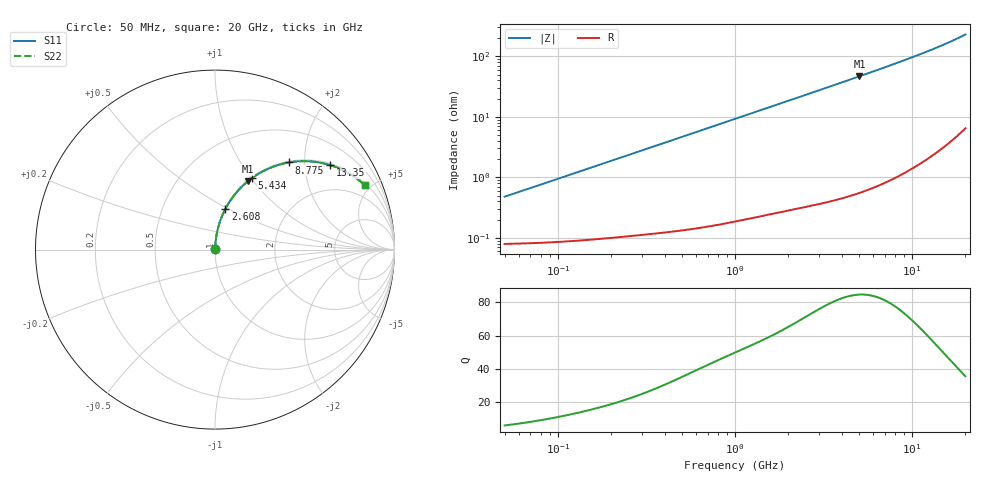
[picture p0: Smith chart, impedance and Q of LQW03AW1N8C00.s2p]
!Murata Part Number: LQW03AW1N8C00
!These Parameters are Measured in Series Mode Connection
!  o--[Z]--o
!Port1  Port2
!  o-------o
!Freq. Start=50[MHz] Stop=20[GHz], 401[Steps]
# Hz S RI R 50
!Freq.(Hz) S11(Real) S11(Imag) S21(Real) S21(Imag) S12(Real) S12(Imag) S22(Real) S22(Imag)
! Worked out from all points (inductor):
!   401 points, 50 MHz to 20 GHz, reference 50 ohm
!   read as one part in series: L = 1.5 nH near 51.52 MHz
!   highest Q = 84.6 at 5.041 GHz (marker M1), where L = 1.48 nH
!   S11 on the Smith chart (normalised r, x): 50 MHz: 1.00, +0.01; 2.608 GHz: 1.01, +0.48; 5.434 GHz: 1.01, +1.01; 8.775 GHz: 1.02, +1.67; 13.35 GHz: 1.05, +2.69; 20 GHz: 1.13, +4.60
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5e7  0.000816 0.00472  0.9992 -0.00472  0.9992 -0.00472  0.000816 0.00472
5.30873e7  0.000822 0.00501  0.9992 -0.00501  0.9992 -0.00501  0.000822 0.00501
1.364002e8  0.00107 0.0128  0.9989 -0.0128  0.9989 -0.0128  0.00107 0.0128
3.721004e8  0.00239 0.0345  0.9976 -0.0345  0.9976 -0.0345  0.00239 0.0345
6.285508e8  0.00483 0.0579  0.9952 -0.0579  0.9952 -0.0579  0.00483 0.0579
1e9  0.0103 0.0914  0.9897 -0.0914  0.9897 -0.0914  0.0103 0.0914
1.639343e9  0.0247 0.147  0.9753 -0.147  0.9753 -0.147  0.0247 0.147
2.608132e9  0.0573 0.2257  0.9427 -0.2257  0.9427 -0.2257  0.0573 0.2257
2.728004e9  0.0622 0.2348  0.9378 -0.2348  0.9378 -0.2348  0.0622 0.2348
3.792786e9  0.1122 0.3095  0.8878 -0.3095  0.8878 -0.3095  0.1122 0.3095
4.405649e9  0.1454 0.3466  0.8546 -0.3466  0.8546 -0.3466  0.1454 0.3466
5.041459e9  0.1823 0.3803  0.8177 -0.3803  0.8177 -0.3803  0.1823 0.3803
5.433528e9  0.206 0.3986  0.794 -0.3986  0.794 -0.3986  0.206 0.3986
6.311513e9  0.2605 0.4329  0.7395 -0.4329  0.7395 -0.4329  0.2605 0.4329
7.442007e9  0.3313 0.4645  0.6687 -0.4645  0.6687 -0.4645  0.3313 0.4645
8.774992e9  0.4123 0.4856  0.5877 -0.4856  0.5877 -0.4856  0.4123 0.4856
1.082228e10  0.5254 0.4918  0.4746 -0.4918  0.4746 -0.4918  0.5254 0.4918
1.334722e10  0.6409 0.4708  0.3591 -0.4708  0.3591 -0.4708  0.6409 0.4708
1.504638e10  0.704 0.4465  0.296 -0.4465  0.296 -0.4465  0.704 0.4465
1.696185e10  0.7628 0.4141  0.2372 -0.4141  0.2372 -0.4141  0.7628 0.4141
1.940974e10  0.822 0.3692  0.178 -0.3692  0.178 -0.3692  0.822 0.3692
2e10  0.8341 0.3582  0.1659 -0.3582  0.1659 -0.3582  0.8341 0.3582
